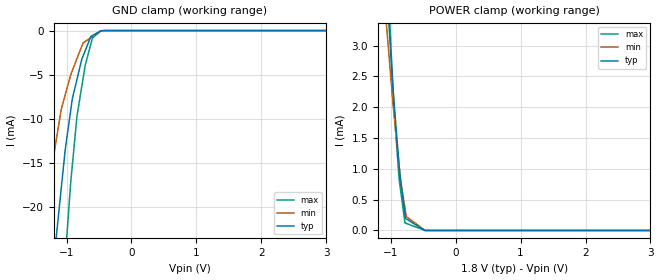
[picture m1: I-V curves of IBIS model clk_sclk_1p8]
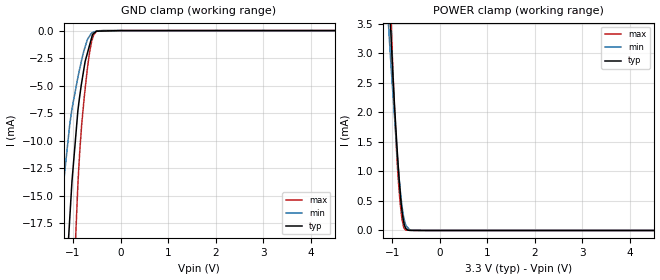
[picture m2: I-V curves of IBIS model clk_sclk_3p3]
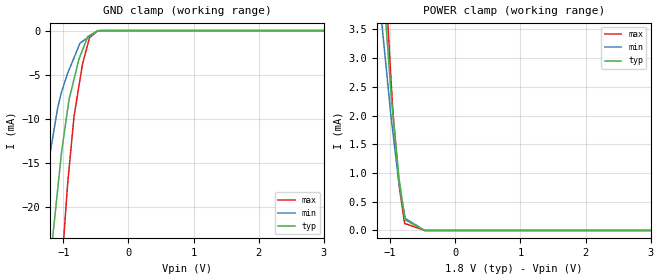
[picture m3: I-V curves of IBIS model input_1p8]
|Texas Instruments Incorporated
|Ultra High Resolution Delta Sigma ADC with PGA for Seismic and Energy
|Exploration
| Marketing part#   Digital Voltage Range   Package-type   #pins
| ADS1282IPW   1.65V to 3.6V   TSSOP   28
| ADS1282IPWG4   1.65V to 3.6V   TSSOP   28
| ADS1282IPWR   1.65V to 3.6V   TSSOP   28
| ADS1282IPWRG4   1.65V to 3.6V   TSSOP   28
[IBIS Ver]   3.2
[File name]   ads1282.ibs
|SIMDE Ver   V2.2 - 201009 - RHL4 - Build 424
[File Rev]   1.0
[Date]   2/21/2011
[Source]
| Texas Instruments Incorporated.
| Analog-eLab Design Center, HPA
| 12500 TI Blvd
| Dallas, TX -75243
| e-mail: elab_ibis@list.ti.com
[Notes]   Revision History:
| Rev 1.0: 2/21/2011
| - Initial version of the model
| - Model generated from simulations in TISPICE
| - Model matched to SPICE simulation
| - C_comp although listed in numerical order of value are
|   obtained from varying PVT conditions. For PVT conditions for
|   each specific value refer the buffer description under
|   respective [Model]. IBIS model user is responsible for using
|   appropriate C_comp to simulate for Signal Integrity.
| - Model names with a trailing _1p8 contains the model for
|   1.8V [1.71V and 1.89V].Model names with a trailing _3p3 contains
|   the model for 3.3V [3.0V and 3.6V].
[Disclaimer]
| This model is designed as an aid for customers of Texas Instruments.
| TI and its licensors and suppliers make no warranties, either expressed
| or implied, with respect to this  model, including the warranties of
| merchantability or fitness for a particular purpose. The model is
| provided solely on an "as is" basis. The entire risk as to its quality
| and performance is with the customer.
[Copyright]
 (C) Copyright 2011 Texas Instruments Incorporated.All rights reserved.
|   ADS1282
[Component]   ADS1282
[Manufacturer]   TI
[Package]   |TSSOP-28 package
|   typ   min   max
R_pkg   0.07736   0.05885   0.09315
L_pkg   2.47760nH   1.81197nH   3.49737nH
C_pkg   0.51604pF   0.40792pF   0.73051pF
[Pin]  signal_name   model_name   R_pin   L_pin   C_pin
1   CLK   CLK_SCLK   0.09097   3.47101nH  0.72743pF
2   SCLK   CLK_SCLK   0.08996   3.07790nH  0.65715pF
3   DRDY   DRDY_MFLAG   0.09016   2.53984nH  0.47586pF
4   DOUT   DOUT   0.07223   2.07348nH  0.41367pF
5   DIN   INPUT   0.06268   1.88509nH  0.41283pF
6   DGND   GND   0.05929   1.82027nH  0.40867pF
7   MCLK   IO   0.06006   1.83688nH  0.41021pF
8   M1   IO   0.06735   1.97912nH  0.41903pF
9   M0   IO   0.07899   2.20805nH  0.42935pF
10   SYNC   INPUT   0.06613   1.95616nH  0.41518pF
11   MFLAG   DRDY_MFLAG   0.07354   2.10536nH  0.41412pF
12   DGND   GND   0.09123   2.56989nH  0.47523pF
13   CAPN   TERM   0.09255   3.13882nH  0.65837pF
14   CAPP   TERM   0.09185   3.49737nH  0.72871pF
15   AINP2   TERM   0.08969   3.45434nH  0.72837pF
16   AINN2   TERM   0.08966   3.07907nH  0.66105pF
17   AINP1   TERM   0.09315   2.60798nH  0.48274pF
18   AINN1   TERM   0.07166   2.06779nH  0.41303pF
19   AVDD   POWER   0.03635   1.74069nH  0.45648pF
20   AVSS   GND   0.03170   1.53782nH  0.45428pF
21   VREFN   TERM   0.05885   1.81197nH  0.41351pF
22   VREFP   TERM   0.07014   2.02800nH  0.42208pF
23   PWDN   INPUT   0.05943   1.82322nH  0.40792pF
24   RESET   INPUT   0.06555   1.94006nH  0.41569pF
25   DGND   GND   0.07223   2.07364nH  0.41326pF
26   DVDD   POWER   0.08964   2.52953nH  0.47709pF
27   DGND   GND   0.08829   3.04259nH  0.66036pF
28   BYPAS   TERM   0.08989   3.44816nH  0.73051pF
|   Model Selectors
[Model Selector] CLK_SCLK
clk_sclk_1p8  1.8V digital input
clk_sclk_3p3  3.3V digital input
[Model Selector] INPUT
input_1p8   1.8V digital input
input_3p3   3.3V digital input
[Model Selector] DOUT
dout_1p8   1.8V 3-state digital output
dout_3p3   3.3V 3-state digital output
[Model Selector] DRDY_MFLAG
drdy_mflag_1p8   1.8V digital output
drdy_mflag_3p3   3.3V digital output
[Model Selector] IO
io_1p8   1.8V digital io
io_3p3   3.3V digital io
[Model Selector] TERM
TERM_1p8  1.8V nominal termination
TERM_3p3  3.3V nominal termination
[Model]  TERM_1p8
Model_type Terminator
C_comp   1.0e-20F  1.0e-20F  1.0e-20F
|   typ   min   max
[Voltage Range]   1.8V   1.71V   1.89V
[POWER Clamp Reference]   1.8V   1.71V   1.89V
[GND Clamp Reference]   0V   0V   0V
|Ambient Temperature   25   85   -40
|Junction Temperature
[Temperature Range]   25   85   -40
[Model]  TERM_3p3
Model_type Terminator
C_comp   1.0e-20F  1.0e-20F  1.0e-20F
|   typ   min   max
[Voltage Range]   3.3V   3.0V   3.6V
[POWER Clamp Reference]   3.3V   3.0V   3.6V
[GND Clamp Reference]   0V   0V   0V
|Ambient Temperature   25   85   -40
|Junction Temperature
[Temperature Range]   25   85   -40
| Models and submodels in the file (12): clk_sclk_1p8 (Input), clk_sclk_3p3 (Input), input_1p8 (Input), input_3p3 (Input), dout_1p8 (3-state), dout_3p3 (3-state), drdy_mflag_1p8 (Output), drdy_mflag_3p3 (Output), io_1p8 (I/O), io_3p3 (I/O), TERM_1p8 (Terminator), TERM_3p3 (Terminator)
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|   clk_sclk_1p8 Model
[Model]   clk_sclk_1p8
Model_type   Input
Vinl = 0.36
Vinh = 1.44
|   typ   min   max
|   (nom PVT)   (Fast PVT)   (slow PVT)
|C_comp from frequency sweep method(F=4.1MHz)
|Average
|C_comp   3.797e-12   3.098e-12   4.604e-12
|C_comp from LC tank measurement(L=1nH)
|Resonant Frequency(Hz)   3.570e+09   3.620e+09   3.430e+09
C_comp   1.989e-12   1.935e-12   2.155e-12
| Where nom  PVT is Nominal Process,  1.8V,  25C
|   Fast PVT is Strong Process,   1.89V,  -40C
|   Slow PVT is Weak Process,   1.71V,  85C
[Model Spec]
Vinl   0.36   0.342   0.378
Vinh   1.44   1.368   1.512
[Voltage Range]   1.8   1.71   1.89
|Ambient Temperature   25   85   -40
|Junction Temperature
[Temperature Range]   25   85   -40
[Power Clamp Reference]   1.8   1.71   1.89
[GND Clamp Reference]   0   0   0
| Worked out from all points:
|   GND clamp passes 1 mA (typ) near -0.64 V on its own axis
|   POWER clamp passes 1 mA (typ) near -0.87 V on its own axis
[GND Clamp]
|   Voltage   I(typ)   I(min)   I(max)
-1.8V     -84.13mA   -48.47mA   -124.1mA
-1.37V    -41.6mA    -22.05mA   -68.55mA
-1.172V   -24.42mA   -13.04mA   -43.36mA
-1.082V   -17.99mA   -8.965mA   -32.87mA
-1.019V   -13.44mA   -7.255mA   -25.7mA
-910.8mV  -7.743mA   -4.549mA   -15.31mA
-839.2mV  -5.545mA   -3.185mA   -9.717mA
-765mV    -3.269mA   -1.773mA   -6.338mA
-714.4mV  -2.317mA   -1.246mA   -4.034mA
-601mV    -571.7uA   -676uA     -846.9uA
-471.6mV  -21.12uA   -25.13uA   -32.35uA
3.6V      0A         0A         0A
[POWER Clamp]
|   Voltage   I(typ)   I(min)   I(max)
-1.8V     20.03mA    16.24mA    24.39mA
-1.084V   4.309mA    3.572mA    5.001mA
-1.049V   3.718mA    3.129mA    4.121mA
-973.8mV  2.436mA    2.169mA    2.496mA
-948.8mV  2.095mA    1.884mA    1.968mA
-869.4mV  1.033mA    1.046mA    824.7uA
-846.5mV  810.1uA    804.1uA    643.5uA
-780.6mV  264.4uA    366uA      123.2uA
-772.2mV  195.1uA    310.4uA    119.9uA
-759.2mV  186.7uA    224.2uA    114.7uA
-470.3mV  3.154nA    52.91nA    107pA
3.6V      0A         0A         0A
|   clk_sclk_3p3 Model
[Model]   clk_sclk_3p3
Model_type   Input
Vinl = 0.66
Vinh = 2.64
|   typ   min   max
|   (nom PVT)   (Fast PVT)   (slow PVT)
|C_comp from frequency sweep method(F=4.1MHz)
|Average
|C_comp   3.879e-12   3.138e-12   4.645e-12
|C_comp from LC tank measurement(L=1nH)
|Resonant Frequency(Hz)   3.470e+09   3.465e+09   3.420e+09
C_comp   2.106e-12   2.105e-12   2.168e-12
| Where nom  PVT is Nominal Process,  3.3V,  25C
|   Fast PVT is Strong Process,   3.6V,  -40C
|   Slow PVT is Weak Process,   3V,  85C
[Model Spec]
Vinl   0.66   0.6   0.72
Vinh   2.64   2.4   2.88
[Voltage Range]   3.3   3   3.6
|Ambient Temperature   25   85   -40
|Junction Temperature
[Temperature Range]   25   85   -40
[Power Clamp Reference]   3.3   3   3.6
[GND Clamp Reference]   0   0   0
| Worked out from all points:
|   GND clamp passes 1 mA (typ) near -0.63 V on its own axis
|   POWER clamp passes 1 mA (typ) near -0.87 V on its own axis
[GND Clamp]
|   Voltage   I(typ)   I(min)   I(max)
-3.3V     -248mA     -170.1mA   -318.9mA
-1.325V   -37.58mA   -19.94mA   -62.38mA
-1.181V   -25.19mA   -13.1mA    -44.73mA
-1.068V   -16.97mA   -8.48mA    -31.17mA
-1.023V   -13.71mA   -7.11mA    -26.59mA
-897.6mV  -7.238mA   -4.229mA   -13.95mA
-864.6mV  -6.101mA   -3.572mA   -11.4mA
-817.2mV  -4.684mA   -2.643mA   -8.505mA
-702mV    -2.116mA   -857.7uA   -3.58mA
-591mV    -361.8uA   -177.7uA   -729uA
-360mV    -38.83uA   -918.3nA   -511.2nA
6.6V      0A         0A         0A
[POWER Clamp]
|   Voltage   I(typ)   I(min)   I(max)
-3.3V     53.29mA    44.99mA    64.35mA
-1.134V   5.379mA    4.241mA    6.245mA
-1.059V   3.861mA    3.227mA    4.425mA
-1.02V    3.201mA    2.726mA    3.468mA
-950.4mV  2.095mA    1.915mA    1.999mA
-896.4mV  1.365mA    1.295mA    1.15mA
-871.2mV  1.057mA    1.043mA    844.7uA
-795.6mV  342.7uA    418.8uA    197.1uA
-745.8mV  93.48uA    179.2uA    34.25uA
-712.8mV  31.29uA    88.73uA    6.698uA
-591mV    1.174uA    2.59uA     2.697uA
6.6V      0A         0A         0A
|   input_1p8 Model
[Model]   input_1p8
Model_type   Input
Vinl = 0.36
Vinh = 1.44
|   typ   min   max
|   (nom PVT)   (Fast PVT)   (slow PVT)
|C_comp from frequency sweep method (F=4.1MHz)
|C_comp   4.062e-12   3.253e-12   4.881e-12
|C_comp from LC tank measurement(L=1nH)
|Resonant Frequency(Hz)   3.510e+09   3.540e+09   3.410e+09
C_comp   2.058e-12   2.023e-12   2.181e-12
| Where nom  PVT is Nominal Process,  1.8V,  25C
|   Fast PVT is Strong Process,   1.89V,  -40C
|   Slow PVT is Weak Process,   1.71V,  85C
[Model Spec]
Vinl   0.36   0.342   0.378
Vinh   1.44   1.368   1.512
[Voltage Range]   1.8   1.71   1.89
|Ambient Temperature   25   85   -40
|Junction Temperature
[Temperature Range]   25   85   -40
[Power Clamp Reference]   1.8   1.71   1.89
[GND Clamp Reference]   0   0   0
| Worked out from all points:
|   GND clamp passes 1 mA (typ) near -0.64 V on its own axis
|   POWER clamp passes 1 mA (typ) near -0.87 V on its own axis
[GND Clamp]
|   Voltage   I(typ)   I(min)   I(max)
-1.8V     -82.42mA   -47mA      -122.1mA
-1.371V   -40.86mA   -21.33mA   -67.88mA
-1.177V   -24.37mA   -12.76mA   -43.86mA
-1.086V   -17.92mA   -8.722mA   -33.25mA
-1.024V   -13.6mA    -6.876mA   -26.64mA
-933.7mV  -8.91mA    -4.843mA   -17.38mA
-912.6mV  -7.82mA    -4.463mA   -15.7mA
-835.4mV  -5.501mA   -3.071mA   -9.725mA
-706.9mV  -2.23mA    -1.231mA   -3.847mA
-597.2mV  -553uA     -669.3uA   -803.8uA
-471.6mV  -21.79uA   -25.86uA   -32.75uA
3.6V      0A         0A         0A
[POWER Clamp]
|   Voltage   I(typ)   I(min)   I(max)
-1.8V     18.18mA    14.63mA    22.22mA
-1.134V   4.776mA    3.67mA     5.787mA
-1.096V   4.087mA    3.238mA    4.912mA
-1.055V   3.44mA     2.759mA    3.99mA
-990.1mV  2.435mA    2.016mA    2.677mA
-981mV    2.301mA    1.925mA    2.496mA
-950.7mV  1.94mA     1.635mA    1.962mA
-863.7mV  906.4uA    803.7uA    793.6uA
-778.7mV  247.9uA    267.9uA    123.3uA
-770.4mV  184.4uA    216.4uA    120uA
-470.3mV  7.13nA     58.45nA    0A
3.6V      0A         0A         0A
